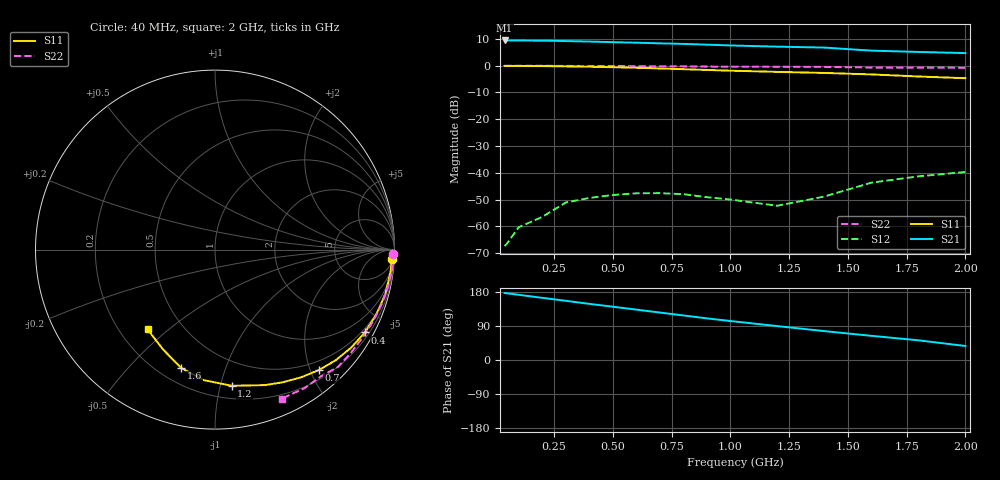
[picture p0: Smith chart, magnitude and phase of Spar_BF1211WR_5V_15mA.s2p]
! NXP part number: BF1212WR
! Bias: VDS = 5V; ID = 15mA; VG1S-start = 0.5V; VG2S = 4V.
! Measured at 2005-04-15 at 14:06:51
#  MHz  S  MA  R 50
! Freq  S11  S21  S12  S22  :
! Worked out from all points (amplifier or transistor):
!   17 points, 40 MHz to 2 GHz, reference 50 ohm
!   highest |S21| = 9.4 dB at 40 MHz (marker M1)
!   |S21| within 3 dB of that: start of sweep to 1.459 GHz
!   unconditionally stable (mu >= 1): 817.8 MHz to end of sweep
!   at 100 MHz: K = 0.12, MSG = 34.9 dB, |S12| = -60.3 dB
!   at 700 MHz: K = 0.67, MSG = 28.0 dB, |S12| = -47.6 dB
!   at 2 GHz: K = 2.94, MAG = 14.6 dB, |S12| = -39.7 dB
!   lowest NFmin = 0.90 dB at 400 MHz
!   S11 on the Smith chart (normalised r, x): 40 MHz: 9, -36; 400 MHz: 0.37, -3.84; 700 MHz: 0.34, -2.13; 1.2 GHz: 0.30, -1.08; 1.6 GHz: 0.29, -0.71; 2 GHz: 0.32, -0.43
40  0.9875 -3.0  2.951 176.8  0.000426 87.8  0.9931 -1.3
50  0.9874 -3.7  2.95 176.0  0.000477 86.0  0.993 -1.6
100  0.9858 -7.4  2.944 172.0  0.000962 84.6  0.9926 -3.1
200  0.9806 -14.7  2.923 164.0  0.001499 90.4  0.993 -6.3
300  0.9689 -21.9  2.875 156.2  0.002781 77.6  0.9882 -9.4
400  0.9541 -28.9  2.814 148.2  0.003384 73.7  0.9852 -12.4
500  0.9345 -35.8  2.742 140.6  0.003843 71.4  0.9812 -15.5
600  0.9122 -42.6  2.681 132.9  0.004135 68.8  0.9764 -18.6
700  0.8858 -49.3  2.607 125.2  0.004157 67.2  0.9712 -21.6
800  0.8579 -56.1  2.543 117.6  0.003983 67.3  0.966 -24.7
900  0.8303 -62.9  2.464 109.9  0.0035 69.2  0.9609 -27.8
1000  0.8047 -69.8  2.38 102.9  0.003163 76.4  0.957 -30.9
1200  0.7644 -83.0  2.262 89.5  0.00242 110.0  0.951 -37.3
1400  0.73 -94.9  2.171 76.2  0.003601 154.0  0.9473 -43.6
1600  0.6856 -106.0  1.904 63.8  0.006527 164.8  0.9204 -50.0
1800  0.6271 -117.5  1.801 52.0  0.008564 175.9  0.9192 -57.1
2000  0.582 -130.2  1.714 37.0  0.01034 -177.3  0.9095 -65.8
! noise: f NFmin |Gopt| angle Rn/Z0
400  0.9  0.693  16.75  29.85
800  1.3  0.707  37.33  29.9
